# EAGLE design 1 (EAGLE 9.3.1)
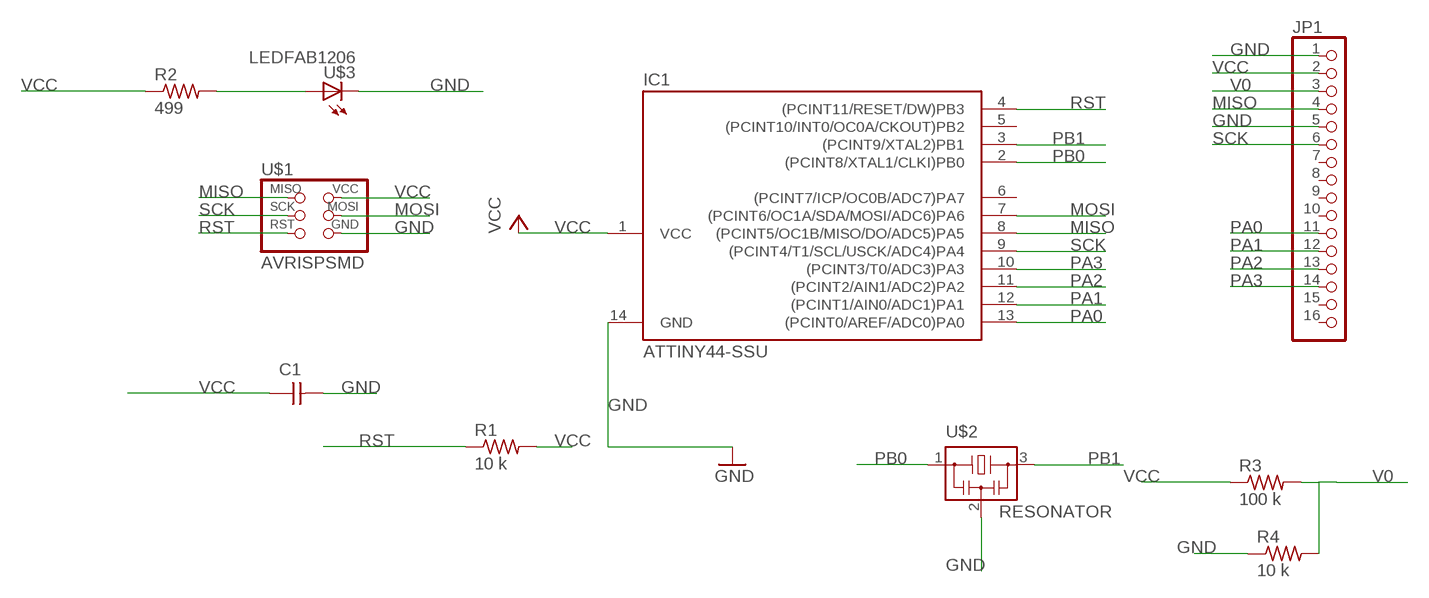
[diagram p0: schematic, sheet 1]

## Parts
C1  CAP-UNPOLARIZEDFAB  [C1206FAB]
IC1  ATTINY44-SSU  [SOIC14]
JP1  PINHD-1X16  [1X16]
R1  10 k  RES-US1206FAB  [R1206FAB]
R2  499  RES-US1206FAB  [R1206FAB]
R3  100 k  RES-US1206FAB  [R1206FAB]
R4  10 k  RES-US1206FAB  [R1206FAB]
U$1  AVRISPSMD  [2X03SMD]
U$2  RESONATOR  [EFOBM]
U$3  LEDFAB1206  [LED1206FAB]

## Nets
GND: C1.2 IC1.14(GND) JP1.1 JP1.5 R4.1 U$1.6(GND) U$2.2 U$3.2(C)
MISO: IC1.8((PCINT5/OC1B/MISO/DO/ADC5)PA5) JP1.4 U$1.1(MISO)
MOSI: IC1.7((PCINT6/OC1A/SDA/MOSI/ADC6)PA6) U$1.4(MOSI)
N$2: R2.2 U$3.1(A)
PA0: IC1.13((PCINT0/AREF/ADC0)PA0) JP1.11
PA1: IC1.12((PCINT1/AIN0/ADC1)PA1) JP1.12
PA2: IC1.11((PCINT2/AIN1/ADC2)PA2) JP1.13
PA3: IC1.10((PCINT3/T0/ADC3)PA3) JP1.14
PB0: IC1.2((PCINT8/XTAL1/CLKI)PB0) U$2.1
PB1: IC1.3((PCINT9/XTAL2)PB1) U$2.3
RST: IC1.4((PCINT11/RESET/DW)PB3) R1.1 U$1.5(RST)
SCK: IC1.9((PCINT4/T1/SCL/USCK/ADC4)PA4) JP1.6 U$1.3(SCK)
V0: JP1.3 R3.2 R4.2
VCC: C1.1 IC1.1(VCC) JP1.2 R1.2 R2.1 R3.1 U$1.2(VCC)
Unconnected: IC1.5((PCINT10/INT0/OC0A/CKOUT)PB2) IC1.6((PCINT7/ICP/OC0B/ADC7)PA7) JP1.7 JP1.8 JP1.9 JP1.10 JP1.15 JP1.16

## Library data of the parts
C1 = fab:CAP-UNPOLARIZED
IC1 = fab:ATTINY44
JP1 = pinhead:PINHD-1X16: PIN HEADER
R1-R4 = fab:RES-US: Resistor (US Symbol)
U$1 = fab:AVRISP
U$2 = fab:RESONATOR
U$3 = fab:LED: LED

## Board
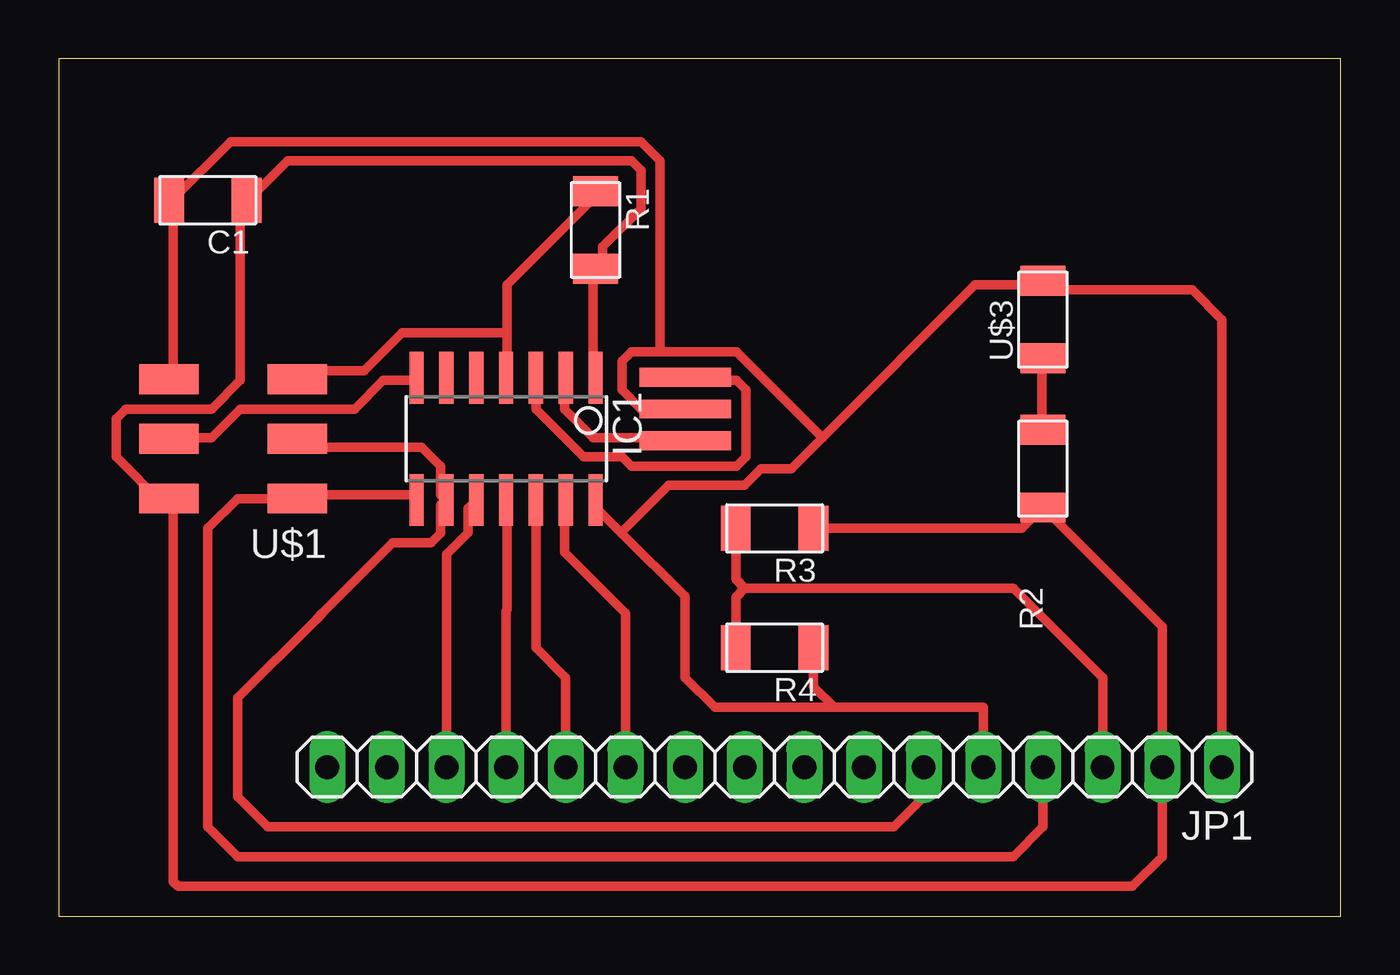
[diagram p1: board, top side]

Size 54.59 x 36.5 mm. Coordinates in mm from the lower left corner, seen from the top.
Outline: 0,0 54.59,0 54.59,36.5 0,36.5 0,0
Copper layers (1*16): Top 0.035mm / dielectric 1.5mm / Bottom 0.035mm
Design rules "default *": minimum track width 16mil, minimum drill 0.35mm, track to track 16mil, track to pad 16mil, pad to pad 16mil, via to via 16mil, smd to smd 16mil, copper to edge 40mil, drill to drill 6mil, minimum pad ring 10mil, minimum via ring 8mil, stop-mask expansion 4mil, vias tented up to drill 0mil, thermal gap 10mil

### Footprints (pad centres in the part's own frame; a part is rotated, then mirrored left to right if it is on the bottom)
C1206FAB = smd 1.27 x 1.905: 1 -1.651,0; 2 1.651,0
SOIC14 = smd 0.61 x 2.21: 1 -3.81,-2.603; 2 -2.54,-2.603; 3 -1.27,-2.603; 4 0,-2.603; 5 1.27,-2.603; 6 2.54,-2.603; 7 3.81,-2.603; 8 3.81,2.603; 9 2.54,2.603; 10 1.27,2.603; 11 0,2.603; 12 -1.27,2.603; 13 -2.54,2.603; 14 -3.81,2.603
1X16 = drill 1.016 long: 1 -19.05,0; 2 -16.51,0; 3 -13.97,0; 4 -11.43,0; 5 -8.89,0; 6 -6.35,0; 7 -3.81,0; 8 -1.27,0; 9 1.27,0; 10 3.81,0; 11 6.35,0; 12 8.89,0; 13 11.43,0; 14 13.97,0; 15 16.51,0; 16 19.05,0
R1206FAB = smd 1.27 x 1.905: 1 -1.651,0; 2 1.651,0
2X03SMD = smd 2.54 x 1.27: 1 -2.54,2.54; 2 2.92,2.54; 3 -2.54,0; 4 2.92,0; 5 -2.54,-2.54; 6 2.92,-2.54
EFOBM = smd 0.8 x 3.9: 1 -1.35,0; 2 0,0; 3 1.35,0
LED1206FAB = smd 1.27 x 1.905: 1 -1.651,0; 2 1.651,0

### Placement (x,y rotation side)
C1  6.35,30.48 180 top
IC1  19.05,20.32 180 top
JP1  30.48,6.35 180 top
R1  22.86,29.21 270 top
R2  41.91,19.05 90 top
R3  30.48,16.51 180 top
R4  30.48,11.43 180 top
U$1  7.62,20.32 180 top
U$2  26.67,21.59 90 top
U$3  41.91,25.4 90 top

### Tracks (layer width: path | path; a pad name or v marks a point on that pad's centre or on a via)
GND
  Top 0.406: U$1.6 4.88,23.22 4.88,30.12 C1.2 4.88,30.53 7.32,32.97 24.79,32.97 25.6,32.16 25.6,24.03 | IC1.14 22.76,17.53 23.95,16.33 | 32.51,20.37 39.01,26.87 41.86,26.87 U$3.2 | 42.27,26.87 U$3.2 | U$2.2 24.79,21.59 23.98,22.4 23.98,23.62 24.38,24.03 25.6,24.03 | 25.6,24.03 28.85,24.03 32.51,20.37 | U$3.2 42.29,26.67 48.26,26.67 49.53,25.4 JP1.1 | 23.95,16.33 26.67,13.61 26.67,10.16 27.94,8.89 33.02,8.89 | JP1.5 39.37,8.89 33.02,8.89 | 32.51,20.37 31.19,19.05 29.9,19.05 29.19,18.34 25.96,18.34 23.95,16.33 | R4.1 32.13,9.78 33.02,8.89
MISO
  Top 0.406: IC1.8 15.04,17.93 10.16,17.93 U$1.1 7.62,17.78 6.35,16.51 6.35,3.81 7.62,2.54 40.64,2.54 41.91,3.81 JP1.4
MOSI
  Top 0.406: IC1.7 15.04,22.81 13.82,22.81 12.6,21.59 7.72,21.59 6.5,20.37 4.88,20.37 U$1.4
N$2
  Top 0.406: R2.2 41.86,20.78 41.86,23.62 U$3.1
PA0
  Top 0.406: IC1.13 21.54,17.53 21.54,15.49 24.13,12.9 JP1.11
PA1
  Top 0.406: JP1.12 21.59,10.16 20.32,11.43 IC1.12
PA2
  Top 0.406: IC1.11 19.1,17.53 19.1,13.06 19.05,13.01 JP1.13
PA3
  Top 0.406: 17.88,17.53 IC1.10 17.42,17.36 17.42,16.33 16.51,15.41 JP1.14 16.61,6.35
PB0
  Top 0.406: IC1.2 21.54,22.81 21.54,21.59 22.76,20.37 26.42,20.37 U$2.1
PB1
  Top 0.406: IC1.3 20.32,21.59 22.35,19.56 23.98,19.56 24.38,19.15 28.85,19.15 29.26,19.56 29.26,22.4 28.85,22.81 26.82,22.81 U$2.3
RST
  Top 0.406: 19.1,24.84 19.1,23.22 IC1.4 | 19.1,24.84 19.1,26.87 22.76,30.53 R1.1 | 19.1,24.84 14.63,24.84 13.01,23.22 10.16,23.22 U$1.5
SCK
  Top 0.406: U$1.3 10.16,19.96 15.44,19.96 16.26,19.15 16.26,17.93 IC1.9 16.26,17.53 16.26,16.31 15.85,15.9 14.22,15.9 11.23,12.9 10.97,12.65 7.62,9.3 7.62,5.08 8.89,3.81 35.56,3.81 36.83,5.08 JP1.6
V0
  Top 0.406: R3.2 28.83,14.35 29.21,13.97 | JP1.3 44.45,10.16 40.64,13.97 29.21,13.97 | R4.2 28.83,13.59 29.21,13.97
VCC
  Top 0.406: 42.27,17.12 R2.1 | IC1.1 22.76,23.22 22.76,27.28 R1.2 23.17,27.69 23.17,28.5 24.79,30.12 24.79,31.75 24.38,32.16 9.75,32.16 8.13,30.53 C1.1 7.72,30.12 7.72,22.81 6.5,21.59 2.85,21.59 2.44,21.18 2.44,19.56 4.47,17.53 U$1.2 4.88,17.53 4.88,1.47 5.08,1.27 45.72,1.27 46.99,2.54 JP1.2 46.99,12.32 R2.1 | R3.1 41.02,16.51 R2.1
